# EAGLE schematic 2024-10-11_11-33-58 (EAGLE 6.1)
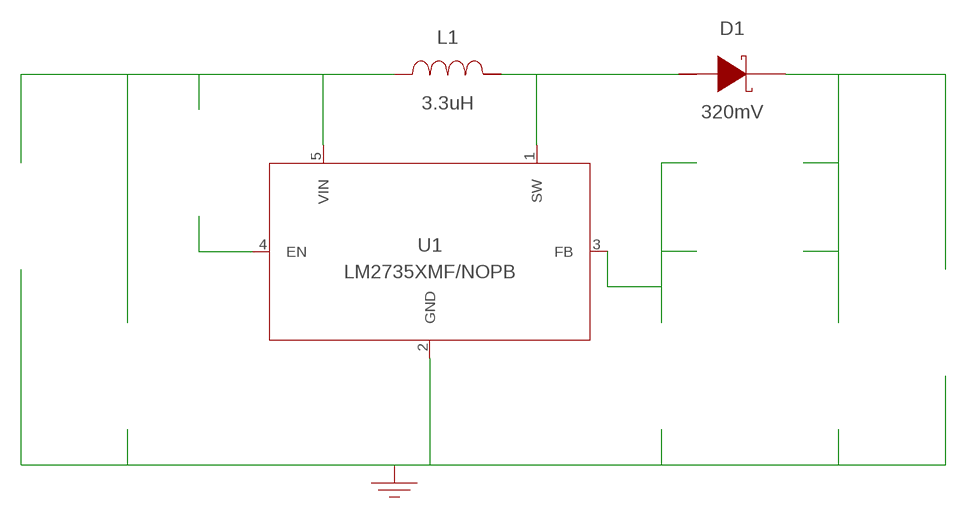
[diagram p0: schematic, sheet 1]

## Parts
CF  1.8nF  CL21C182JBF1PNECL21C182JBF1PNE  [0805]  (not placed on a sheet)
CIN  10uF  C0805C106K8PACTUC0805C106K8PACTU  [0805]  (not placed on a sheet)
COUT  22uF  GRM21BD70J226ME44LGRM21BD70J226ME44L  [0805]  (not placed on a sheet)
D1  320mV  CMS06CMS06  [M-FLAT]
GND  WB_GND  WB_GNDWB_GND  [WB_GND]
IOUT  WB_CURRENT_LOAD  WB_CURRENT_LOADWB_CURRENT_LOAD  [WB_CURRENT_LOAD]  (not placed on a sheet)
L1  3.3uH  SLF7045T-3R3M2R5-PFSLF7045T-3R3M2R5-PF  [SLF7045]
RENABLE  10k  CRCW080510K0FKEACRCW080510K0FKEA  [0805]  (not placed on a sheet)
RFBB  10k  CRCW080510K0FKEACRCW080510K0FKEA  [0805]  (not placed on a sheet)
RFBT  30k  RR1220P-303-DRR1220P-303-D  [0805]  (not placed on a sheet)
U1  LM2735XMF/NOPB  LM2735XMF/NOPBLM2735XMF/NOPB  [MF05A]
VIN  WB_BATTERY  WB_BATTERYWB_BATTERY  [WB_BATTERY]  (not placed on a sheet)
Unconnected: CF.1 CF.2 CIN.1 CIN.2 COUT.1 COUT.2 D1.1(K) D1.2(A) GND.1 IOUT.1(+) IOUT.2(-) L1.1 L1.2 RENABLE.1 RENABLE.2 RFBB.1 RFBB.2 RFBT.1 RFBT.2 U1.1(SW) U1.2(GND) U1.3(FB) U1.4(EN) U1.5(VIN) VIN.1(+) VIN.2(-)

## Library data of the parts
CF = AcceleratedDesigns_Lib:CL21C182JBF1PNE; Manufacturer_Part_Number: CL21C182JBF1PNE; Vendor: Samsung Electro-Mechanics
CIN = AcceleratedDesigns_Lib:C0805C106K8PACTU; Manufacturer_Part_Number: C0805C106K8PACTU; Vendor: Kemet
COUT = AcceleratedDesigns_Lib:GRM21BD70J226ME44L; Manufacturer_Part_Number: GRM21BD70J226ME44L; Vendor: MuRata
D1 = AcceleratedDesigns_Lib:CMS06; Manufacturer_Part_Number: CMS06; Vendor: Toshiba
GND = AcceleratedDesigns_Lib:WB_GND; Manufacturer_Part_Number: WB_GND
IOUT = AcceleratedDesigns_Lib:WB_CURRENT_LOAD; Manufacturer_Part_Number: WB_CURRENT_LOAD
L1 = AcceleratedDesigns_Lib:SLF7045T-3R3M2R5-PF; Manufacturer_Part_Number: SLF7045T-3R3M2R5-PF; Vendor: TDK
RENABLE RFBB = AcceleratedDesigns_Lib:CRCW080510K0FKEA; Manufacturer_Part_Number: CRCW080510K0FKEA; Vendor: Vishay-Dale
RFBT = AcceleratedDesigns_Lib:RR1220P-303-D; Manufacturer_Part_Number: RR1220P-303-D; Vendor: Susumu Co Ltd
U1 = AcceleratedDesigns_Lib:LM2735XMF/NOPB; Manufacturer_Part_Number: LM2735XMF/NOPB; Vendor: Texas Instruments
VIN = AcceleratedDesigns_Lib:WB_BATTERY; Manufacturer_Part_Number: WB_BATTERY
